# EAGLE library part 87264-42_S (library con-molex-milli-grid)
RECEPTACAL
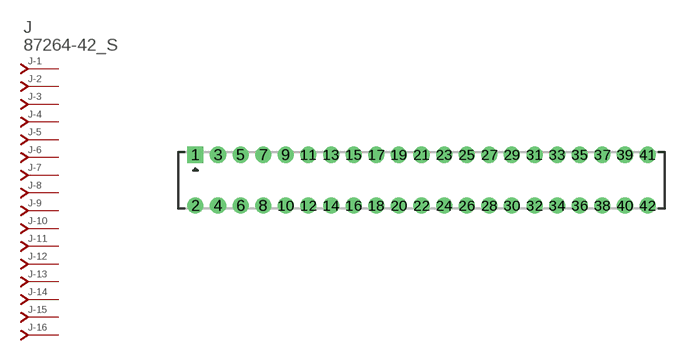
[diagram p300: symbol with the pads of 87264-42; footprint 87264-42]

Designator prefix J; gates -1=J-NV -2=J-N -3=J-N -4=J-N -5=J-N -6=J-N -7=J-N -8=J-N -9=J-N -10=J-N -11=J-N -12=J-N -13=J-N -14=J-N -15=J-N -16=J-N -17=J-N -18=J-N -19=J-N -20=J-N -21=J-N -22=J-N -23=J-N -24=J-N -25=J-N -26=J-N -27=J-N -28=J-N -29=J-N -30=J-N -31=J-N -32=J-N -33=J-N -34=J-N -35=J-N -36=J-N -37=J-N -38=J-N -39=J-N -40=J-N -41=J-N -42=J-N

## 87264-42_S  [87264-42]
1  -1:J  pas
2  -2:J  pas
3  -3:J  pas
4  -4:J  pas
5  -5:J  pas
6  -6:J  pas
7  -7:J  pas
8  -8:J  pas
9  -9:J  pas
10  -10:J  pas
11  -11:J  pas
12  -12:J  pas
13  -13:J  pas
14  -14:J  pas
15  -15:J  pas
16  -16:J  pas
17  -17:J  pas
18  -18:J  pas
19  -19:J  pas
20  -20:J  pas
21  -21:J  pas
22  -22:J  pas
23  -23:J  pas
24  -24:J  pas
25  -25:J  pas
26  -26:J  pas
27  -27:J  pas
28  -28:J  pas
29  -29:J  pas
30  -30:J  pas
31  -31:J  pas
32  -32:J  pas
33  -33:J  pas
34  -34:J  pas
35  -35:J  pas
36  -36:J  pas
37  -37:J  pas
38  -38:J  pas
39  -39:J  pas
40  -40:J  pas
41  -41:J  pas
42  -42:J  pas

## Footprint 87264-42 (pad centres in mm)
RECEPTACAL Dual Row, Side Entry
drill 0.914 square: 1 -20,2.25
drill 0.914: 2 -20,-2.25; 3 -18,2.25; 4 -18,-2.25; 5 -16,2.25; 6 -16,-2.25; 7 -14,2.25; 8 -14,-2.25; 9 -12,2.25; 10 -12,-2.25; 11 -10,2.25; 12 -10,-2.25; 13 -8,2.25; 14 -8,-2.25; 15 -6,2.25; 16 -6,-2.25; 17 -4,2.25; 18 -4,-2.25; 19 -2,2.25; 20 -2,-2.25; 21 0,2.25; 22 0,-2.25; 23 2,2.25; 24 2,-2.25; 25 4,2.25; 26 4,-2.25; 27 6,2.25; 28 6,-2.25; 29 8,2.25; 30 8,-2.25; 31 10,2.25; 32 10,-2.25; 33 12,2.25; 34 12,-2.25; 35 14,2.25; 36 14,-2.25; 37 16,2.25; 38 16,-2.25; 39 18,2.25; 40 18,-2.25; 41 20,2.25; 42 20,-2.25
